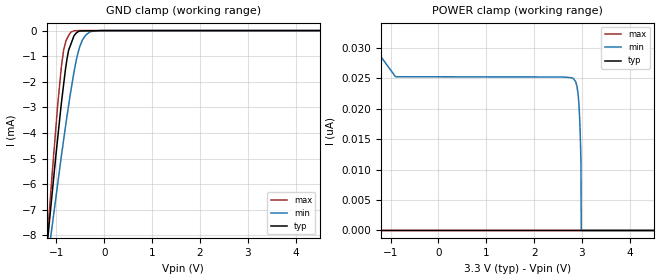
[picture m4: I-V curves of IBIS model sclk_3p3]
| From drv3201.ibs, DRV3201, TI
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|   sclk_3p3 Model
[Model]   sclk_3p3
Model_type   Input
Vinl = 0.99
Vinh = 2.31
|   typ   min   max
|   (nom PVT)   (fast PVT)   (slow PVT)
 C_comp   4.837e-13   4.556e-13   5.145e-13
| Where nom  PVT is Nominal Process, 3.3V, 27C
|   Fast PVT is Strong Process,  3.6V, -40C
|   Slow PVT is Weak Process,   3V, 150C
[Voltage Range]   3.3   3   3.6
|Junction Temperature
[Temperature Range]   27   150   -40
[Power Clamp Reference]   3.3   3   3.6
[GND Clamp Reference]   0   0   0
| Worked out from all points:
|   GND clamp passes 1 mA (typ) near -0.77 V on its own axis
[GND Clamp]
|   Voltage   I(typ)   I(min)   I(max)
-3.3V     -51.87mA   -41.42mA   -64mA
-1.181V   -8.098mA   -8.925mA   -7.863mA
-1.094V   -6.437mA   -7.691mA   -5.696mA
-975.6mV  -4.223mA   -6.005mA   -2.939mA
-896.4mV  -2.815mA   -4.882mA   -1.39mA
-849.6mV  -2.092mA   -4.261mA   -761.1uA
-745.8mV  -765.6uA   -2.918mA   -198.4uA
-633.6mV  -202.4uA   -1.621mA   -5.446uA
-561mV    -57.22uA   -949.5uA   -1.856uA
-456mV    -14.23uA   -362.7uA   0A
-285mV    -8.857uA   -38.16uA   0A
6.6V      0A         0A         0A
[POWER Clamp]
|   Voltage   I(typ)   I(min)   I(max)
-3.3V     39.34uA    36.16uA    41.34uA
-2.482V   1.6uA      4.007uA    92.63nA
-2.462V   1.167uA    3.403uA    0A
-2.334V   79.73nA    551.3nA    0A
-2.32V    10.28nA    501.1nA    0A
-2.19V    0A         39.15nA    0A
-897mV    0A         25.23nA    0A
2.817V    0A         24.95nA    0A
2.943V    0A         19.78nA    0A
2.979V    0A         10.93nA    0A
2.985V    0A         0A         0A
6.6V      0A         0A         0A
